| IBIS file stm32h563_573_lqfp144-smps.ibs
[IBIS ver] 4.2
[File name] stm32h563_573_lqfp144-smps.ibs
[File Rev] 1.1
[Date] 07-05-2024
[Source] Data Created at STMicroelectronics
[Notes]  File originated from ELDO simulations.
[Disclaimer]  This information is for modeling purpose only and is
   not guaranteed. The information is subject to change without
   notice.
[Copyright] Copyright 2024 STMicroelectronics Inc.
|   Component stm32h563_573_lqfp144-smps
[Component] stm32h563_573_lqfp144-smps
[Manufacturer] STMicroelectronics
[Package]
| variable   typ   min   max
R_pkg  0  NA  NA
L_pkg  0  NA  NA
C_pkg  0  NA  NA
[Pin]   signal_name   model_name
1  PE2  io8_ft_i3c_spi
2  PE3  io8_ft_i3c_spi
3  PE4  io8_ft_i3c_spi
4  PE5  io8_ft_i3c_spi
5  PE6  io8_ft_i3c_spi
6  VBAT  power
7  PC13  io8_ft_i3c_spi
8  PC14-OSC32_IN  io8_ft_i3c_spi
9  PC15  io8_ft_i3c_spi
10  PF0  io8_ft_i3c_spi
11  PF1  io8_ft_i3c_spi
12  PF2  io8_ft_i3c_spi
13  PF3  io8_ft_i3c_spi
14  PF4  io8_ft_i3c_spi
15  PF5  io8_ft_i3c_spi
16  VSS  gnd
17  VDD  power
18  PF6  io8_ft_i3c_spi
19  PF7  io8_ft_i3c_spi
20  PF8  io8_ft_i3c_spi
21  PF9  io8_ft_i3c_spi
22  PF10  io8_ft_i3c_spi
23  PH0-OSC_IN  io8_ft_i3c_spi
24  PH1-OSC_OUT  io8_ft_i3c_spi
25  NRST  ioreset_ft_v33
26  PC0  io8_ft_spi
27  PC1  io8_ft_spi
28  PC2  io8_ft_spi
29  PC3  io8_ft_spi
30  VSSA  nc
31  VREFP  nc
32  VDDA  nc
33  PA0  io8_ft_spi
34  PA1  io8_ft_spi_tamp
35  PA2  io8_ft_spi
36  PA3  io8_ft_spi
37  VSS  gnd
38  VDD  power
39  PA4  io8_ft_spi
40  PA5  io8_ft_spi
41  PA6  io8_ft_spi
42  PA7  io8_ft_spi
43  PB0  io8_ft_spi
44  PB1  io8_ft_spi
45  PB2  io8_ft_i3c_spi
46  PF11  io8_ft_spi
47  PF12  io8_ft_spi
48  VSS  gnd
49  VDD  power
50  PF13  io8_ft_spi
51  PF14  io8_ft_spi
52  PF15  io8_ft_i3c_spi
53  PG0  io8_ft_i3c_spi
54  PG1  io8_ft_i3c_spi
55  PE7  io8_ft_i3c_spi
56  PE8  io8_ft_i3c_spi
57  PE9  io8_ft_i3c_spi
58  VSS  gnd
59  VDD  power
60  PE10  io8_ft_i3c_spi
61  PE11  io8_ft_i3c_spi
62  PE12  io8_ft_i3c_spi
63  PE13  io8_ft_i3c_spi
64  PE14  io8_ft_i3c_spi
65  PE15  io8_ft_i3c_spi
66  PB10  io8_ft_i3c_spi
67  PB11  io8_ft_i3c_spi
68  VLXSMPS  nc
69  VDDSMPS  nc
70  VSSSMPS  nc
71  VCAP  nc
72  VSS  gnd
73  VDD  power
|74  PB13  io8usb_ft_pd
|75  PB14  io8usb_ft_pd
74  PB13  nc
75  PB14  nc
76  PB15  io8_ft_spi
77  PD8  io8_ft_i3c_spi
78  PD9  io8_ft_i3c_spi
79  PD10  io8_ft_i3c_spi
80  PD11  io8_ft_i3c_spi
81  PD12  io8_ft_i3c_spi
82  PD13  io8_ft_i3c_spi
83  VSS  gnd
84  VDD  power
85  PD14  io8_ft_i3c_spi
86  PD15  io8_ft_i3c_spi
87  PG2  io8_ft_i3c_spi
88  PG3  io8_ft_i3c_spi
89  PG4  io8_ft_i3c_spi
90  PG5  io8_ft_i3c_spi
91  PG6  io8_ft_i3c_spi
92  PG7  io8_ft_i3c_spi
93  PG8  io8_ft_i3c_spi
94  VSS  gnd
95  VDD  power
96  PC6  io8_ft_i3c_spi
97  PC7  io8_ft_i3c_spi
98  PC8  io8_ft_i3c_spi
99  PC9  io8_ft_i3c_spi
100  PA8  io8_ft_i3c_spi
101  PA9  io8_ft_i3c_spi
102  PA10  io8_ft_i3c_spi
103  PA11  io8usb_ft_i3c_spi_phy
104  PA12  io8usb_ft_i3c_spi_phy
105  PA13  io8_ft_i3c_spi
106  VDDUSB  power
107  VSS  gnd
108  VDD  power
109  PA14  io8_ft_i3c_spi
110  PA15  io8_ft_i3c_spi
111  PC10  io8_ft_i3c_spi
112  PC11  io8_ft_i3c_spi
113  PC12  io8_ft_i3c_spi
114  PD0  io8_ft_i3c_spi
115  PD1  io8_ft_i3c_spi
116  PD2  io8_ft_i3c_spi
117  PD3  io8_ft_i3c_spi
118  PD4  io8_ft_i3c_spi
119  PD5  io8_ft_i3c_spi
120  VSS  gnd
121  VDDIO2  power
122  PD6  io8_ft_i3c_spi
123  PD7  io8_ft_i3c_spi
124  PG9  io8_ft_i3c_spi
125  PG10  io8_ft_i3c_spi
126  PG12  io8_ft_i3c_spi
127  PG13  io8_ft_i3c_spi
128  PG14  io8_ft_i3c_spi
129  VSS  gnd
130  VDD  power
131  PG15  io8_ft_i3c_spi
132  PB3  io8_ft_i3c_spi
133  PB4  io8_ft_i3c_spi
134  PB5  io8_ft_i3c_spi
135  PB6  io8_ft_i3c_spi
136  PB7  io8_ft_i3c_spi
137  BOOT0  vpphv
138  PB8  io8_ft_i3c_spi
139  PB9  io8_ft_i3c_spi
140  PE0  io8_ft_i3c_spi
141  PE1  io8_ft_i3c_spi
142  VCAP  nc
143  VSS  gnd
144  VDD  power
[Package Model]   484-lqfp-20x20-144-smps-221014
[Pin Mapping]   pulldown_ref   pullup_ref   | Comment
1  gndio  vddiom
2  gndio  vddiom
3  gndio  vddiom
4  gndio  vddiom
5  gndio  vddiom
6  nc  vsw
7  gndio  vddiom  | Depending on IO usage
| 7  gndio  vsw  | Depending on IO usage
8  gndio  vddiom  | Depending on IO usage
| 8  gndio  vsw  | Depending on IO usage
9  gndio  vddiom  | Depending on IO usage
| 9  gndio  vsw  | Depending on IO usage
10  gndio  vddiom
11  gndio  vddiom
12  gndio  vddiom
13  gndio  vddiom
14  gndio  vddiom
15  gndio  vddiom
16  gndio  nc
17  nc  vddiom
18  gndio  vddiom
19  gndio  vddiom
20  gndio  vddiom
21  gndio  vddiom
22  gndio  vddiom
23  gndio  vddiom
24  gndio  vddiom
25  gndio  vddiom
26  gndio  vddiom
27  gndio  vddiom
28  gndio  vddiom
29  gndio  vddiom
30  nc  nc
31  nc  nc
32  nc  nc
33  gndio  vddiom
34  gndio  vddiom
35  gndio  vddiom
36  gndio  vddiom
37  gndio  nc
38  nc  vddiom
39  gndio  vddiom
40  gndio  vddiom
41  gndio  vddiom
42  gndio  vddiom
43  gndio  vddiom
44  gndio  vddiom
45  gndio  vddiom
46  gndio  vddiom
47  gndio  vddiom
48  gndio  nc
49  nc  vddiom
50  gndio  vddiom
51  gndio  vddiom
52  gndio  vddiom
53  gndio  vddiom
54  gndio  vddiom
55  gndio  vddiom
56  gndio  vddiom
57  gndio  vddiom
58  gndio  nc
59  nc  vddiom
60  gndio  vddiom
61  gndio  vddiom
62  gndio  vddiom
63  gndio  vddiom
64  gndio  vddiom
65  gndio  vddiom
66  gndio  vddiom
67  gndio  vddiom
68  nc  nc
69  nc  nc
70  nc  nc
71  nc  nc
72  gndio  nc
73  nc  vddiom
|74  gndio  vddiom
|75  gndio  vddiom
74 nc nc
75 nc nc
76  gndio  vddiom
77  gndio  vddiom
78  gndio  vddiom
79  gndio  vddiom
80  gndio  vddiom
81  gndio  vddiom
82  gndio  vddiom
83  gndio  nc
84  nc  vddiom
85  gndio  vddiom
86  gndio  vddiom
87  gndio  vddiom
88  gndio  vddiom
89  gndio  vddiom
90  gndio  vddiom
91  gndio  vddiom
92  gndio  vddiom
93  gndio  vddiom
94  gndio  nc
95  nc  vddiom
96  gndio  vddiom
97  gndio  vddiom
98  gndio  vddiom
99  gndio  vddiom
100  gndio  vddiom
101  gndio  vddiom  | Depending on IO usage
| 101  gndio  vddusb  | Depending on IO usage
102  gndio  vddiom  | Depending on IO usage
| 102  gndio  vddusb  | Depending on IO usage
103  gndio  vddiom  | Depending on IO usage
| 103  gndio  vddusb  | Depending on IO usage
104  gndio  vddiom  | Depending on IO usage
| 104  gndio  vddusb  | Depending on IO usage
105  gndio  vddiom  | Depending on IO usage
| 105  gndio  vddusb  | Depending on IO usage
106  nc  vddusb
107  gndio  nc
108  nc  vddiom
109  gndio  vddiom
110  gndio  vddiom
111  gndio  vddiom
112  gndio  vddiom
113  gndio  vddiom
114  gndio  vddiom
115  gndio  vddiom
116  gndio  vddiom
117  gndio  vddiom
118  gndio  vddiom
119  gndio  vddiom
120  gndio  nc
121  nc  vddmmc
122  gndio  vddiom  | Depending on IO usage
| 122  gndio  vddmmc  | Depending on IO usage
123  gndio  vddiom  | Depending on IO usage
| 123  gndio  vddmmc  | Depending on IO usage
124  gndio  vddiom  | Depending on IO usage
| 124  gndio  vddmmc  | Depending on IO usage
125  gndio  vddiom  | Depending on IO usage
| 125  gndio  vddmmc  | Depending on IO usage
126  gndio  vddiom  | Depending on IO usage
| 126  gndio  vddmmc  | Depending on IO usage
127  gndio  vddiom  | Depending on IO usage
| 127  gndio  vddmmc  | Depending on IO usage
128  gndio  vddiom  | Depending on IO usage
| 128  gndio  vddmmc  | Depending on IO usage
129  gndio  nc
130  nc  vddiom
131  gndio  vddiom  | Depending on IO usage
| 131  gndio  vddmmc  | Depending on IO usage
132  gndio  vddiom  | Depending on IO usage
| 132  gndio  vddmmc  | Depending on IO usage
133  gndio  vddiom  | Depending on IO usage
| 133  gndio  vddmmc  | Depending on IO usage
134  gndio  vddiom  | Depending on IO usage
| 134  gndio  vddmmc  | Depending on IO usage
135  gndio  vddiom  | Depending on IO usage
| 135  gndio  vddmmc  | Depending on IO usage
136  gndio  vddiom  | Depending on IO usage
| 136  gndio  vddmmc  | Depending on IO usage
137  gndio  vddiom  | Depending on IO usage
| 137  gndio  vddmmc  | Depending on IO usage
138  gndio  vddiom  | Depending on IO usage
| 138  gndio  vddmmc  | Depending on IO usage
139  gndio  vddiom  | Depending on IO usage
| 139  gndio  vddmmc  | Depending on IO usage
140  gndio  vddiom  | Depending on IO usage
| 140  gndio  vddmmc  | Depending on IO usage
141  gndio  vddiom  | Depending on IO usage
| 141  gndio  vddmmc  | Depending on IO usage
142  nc  nc
143  gndio  nc
144  nc  vddiom
[Model Selector] io8_ft_i3c_spi
io8_ft_spi_ls_1v2 "io8_ft spi low speed @ 1.2V"
io8_ft_spi_ls_1v8 "io8_ft spi low speed @ 1.8V"
io8_ft_spi_ls_3v3 "io8_ft spi low speed @ 3.3V"
io8_ft_spi_ms_1v2 "io8_ft spi med speed @ 1.2V"
io8_ft_spi_ms_1v8 "io8_ft spi med speed @ 1.8V"
io8_ft_spi_ms_3v3 "io8_ft spi med speed @ 3.3V"
io8_ft_spi_fs_1v2 "io8_ft spi fast speed @ 1.2V"
io8_ft_spi_fs_1v8 "io8_ft spi fast speed @ 1.8V"
io8_ft_spi_fs_3v3 "io8_ft spi fast speed @ 3.3V"
io8_ft_spi_hs_1v2 "io8_ft spi high speed @ 1.2V"
io8_ft_spi_hs_1v8 "io8_ft spi high speed @ 1.8V"
io8_ft_spi_hs_3v3 "io8_ft spi high speed @ 3.3V"
io8_ft_hslv_spi_ls_1v2 "io8_ft spi hslv low speed @ 1.2V"
io8_ft_hslv_spi_ls_1v8 "io8_ft spi hslv low speed @ 1.8V"
io8_ft_hslv_spi_ls_2v5 "io8_ft spi hslv low speed @ 2.5V"
io8_ft_hslv_spi_ms_1v2 "io8_ft spi hslv med speed @ 1.2V"
io8_ft_hslv_spi_ms_1v8 "io8_ft spi hslv med speed @ 1.8V"
io8_ft_hslv_spi_ms_2v5 "io8_ft spi hslv med speed @ 2.5V"
io8_ft_hslv_spi_fs_1v2 "io8_ft spi hslv fast speed @ 1.2V"
io8_ft_hslv_spi_fs_1v8 "io8_ft spi hslv fast speed @ 1.8V"
io8_ft_hslv_spi_fs_2v5 "io8_ft spi hslv fast speed @ 2.5V"
io8_ft_hslv_spi_hs_1v2 "io8_ft spi hslv high speed @ 1.2V"
io8_ft_hslv_spi_hs_1v8 "io8_ft spi hslv high speed @ 1.8V"
io8_ft_hslv_spi_hs_2v5 "io8_ft spi hslv high speed @ 2.5V"
io8_ft_i3c_spi_ls_1v2 "io8_ft i3c spi open-drain low speed @ 1.2V"
io8_ft_i3c_spi_ls_1v8 "io8_ft i3c spi open-drain low speed @ 1.8V"
io8_ft_i3c_spi_ls_3v3 "io8_ft i3c spi open-drain low speed @ 3.3V"
io8_ft_i3c_spi_ms_1v2 "io8_ft i3c spi open-drain med speed @ 1.2V"
io8_ft_i3c_spi_ms_1v8 "io8_ft i3c spi open-drain med speed @ 1.8V"
io8_ft_i3c_spi_ms_3v3 "io8_ft i3c spi open-drain med speed @ 3.3V"
io8_ft_i3c_spi_fs_1v2 "io8_ft i3c spi open-drain fast speed @ 1.2V"
io8_ft_i3c_spi_fs_1v8 "io8_ft i3c spi open-drain fast speed @ 1.8V"
io8_ft_i3c_spi_fs_3v3 "io8_ft i3c spi open-drain fast speed @ 3.3V"
io8_ft_i3c_spi_hs_1v2 "io8_ft i3c spi open-drain high speed @ 1.2V"
io8_ft_i3c_spi_hs_1v8 "io8_ft i3c spi open-drain high speed @ 1.8V"
io8_ft_i3c_spi_hs_3v3 "io8_ft i3c spi open-drain high speed @ 3.3V"
io8_ft_hslv_i3c_spi_ls_1v2 "io8_ft hslv i3c spi open-drain low speed @ 1.2V"
io8_ft_hslv_i3c_spi_ls_1v8 "io8_ft hslv i3c spi open-drain low speed @ 1.8V"
io8_ft_hslv_i3c_spi_ls_2v5 "io8_ft hslv i3c spi open-drain low speed @ 2.5V"
io8_ft_hslv_i3c_spi_ms_1v2 "io8_ft hslv i3c spi open-drain med speed @ 1.2V"
io8_ft_hslv_i3c_spi_ms_1v8 "io8_ft hslv i3c spi open-drain med speed @ 1.8V"
io8_ft_hslv_i3c_spi_ms_2v5 "io8_ft hslv i3c spi open-drain med speed @ 2.5V"
io8_ft_hslv_i3c_spi_fs_1v2 "io8_ft hslv i3c spi open-drain fast speed @ 1.2V"
io8_ft_hslv_i3c_spi_fs_1v8 "io8_ft hslv i3c spi open-drain fast speed @ 1.8V"
io8_ft_hslv_i3c_spi_fs_2v5 "io8_ft hslv i3c spi open-drain fast speed @ 2.5V"
io8_ft_hslv_i3c_spi_hs_1v2 "io8_ft hslv i3c spi open-drain high speed @ 1.2V"
io8_ft_hslv_i3c_spi_hs_1v8 "io8_ft hslv i3c spi open-drain high speed @ 1.8V"
io8_ft_hslv_i3c_spi_hs_2v5 "io8_ft hslv i3c spi open-drain high speed @ 2.5V"
io8_ft_i3c_fmp_spi_3v3 "io8_ft i3c fm+ spi open-drain @ 3.3V"
io8_ft_i3c_fmp_spi_1v8 "io8_ft i3c fm+ spi open-drain @ 1.8V"
io8_ft_i3c_fmp_spi_1v2 "io8_ft i3c fm+ spi open-drain @ 1.2V"
[Model Selector] io8_ft_spi
io8_ft_spi_ls_1v2 "io8_ft spi low speed @ 1.2V"
io8_ft_spi_ls_1v8 "io8_ft spi low speed @ 1.8V"
io8_ft_spi_ls_3v3 "io8_ft spi low speed @ 3.3V"
io8_ft_spi_ms_1v2 "io8_ft spi med speed @ 1.2V"
io8_ft_spi_ms_1v8 "io8_ft spi med speed @ 1.8V"
io8_ft_spi_ms_3v3 "io8_ft spi med speed @ 3.3V"
io8_ft_spi_fs_1v2 "io8_ft spi fast speed @ 1.2V"
io8_ft_spi_fs_1v8 "io8_ft spi fast speed @ 1.8V"
io8_ft_spi_fs_3v3 "io8_ft spi fast speed @ 3.3V"
io8_ft_spi_hs_1v2 "io8_ft spi high speed @ 1.2V"
io8_ft_spi_hs_1v8 "io8_ft spi high speed @ 1.8V"
io8_ft_spi_hs_3v3 "io8_ft spi high speed @ 3.3V"
io8_ft_hslv_spi_ls_1v2 "io8_ft spi hslv low speed @ 1.2V"
io8_ft_hslv_spi_ls_1v8 "io8_ft spi hslv low speed @ 1.8V"
io8_ft_hslv_spi_ls_2v5 "io8_ft spi hslv low speed @ 2.5V"
io8_ft_hslv_spi_ms_1v2 "io8_ft spi hslv med speed @ 1.2V"
io8_ft_hslv_spi_ms_1v8 "io8_ft spi hslv med speed @ 1.8V"
io8_ft_hslv_spi_ms_2v5 "io8_ft spi hslv med speed @ 2.5V"
io8_ft_hslv_spi_fs_1v2 "io8_ft spi hslv fast speed @ 1.2V"
io8_ft_hslv_spi_fs_1v8 "io8_ft spi hslv fast speed @ 1.8V"
io8_ft_hslv_spi_fs_2v5 "io8_ft spi hslv fast speed @ 2.5V"
io8_ft_hslv_spi_hs_1v2 "io8_ft spi hslv high speed @ 1.2V"
io8_ft_hslv_spi_hs_1v8 "io8_ft spi hslv high speed @ 1.8V"
io8_ft_hslv_spi_hs_2v5 "io8_ft spi hslv high speed @ 2.5V"
[Model Selector] io8_ft_spi_tamp
io8_ft_spi_ls_1v2 "io8_ft spi low speed @ 1.2V"
io8_ft_spi_ls_1v8 "io8_ft spi low speed @ 1.8V"
io8_ft_spi_ls_3v3 "io8_ft spi low speed @ 3.3V"
io8_ft_spi_ms_1v2 "io8_ft spi med speed @ 1.2V"
io8_ft_spi_ms_1v8 "io8_ft spi med speed @ 1.8V"
io8_ft_spi_ms_3v3 "io8_ft spi med speed @ 3.3V"
io8_ft_spi_fs_1v2 "io8_ft spi fast speed @ 1.2V"
io8_ft_spi_fs_1v8 "io8_ft spi fast speed @ 1.8V"
io8_ft_spi_fs_3v3 "io8_ft spi fast speed @ 3.3V"
io8_ft_spi_hs_1v2 "io8_ft spi high speed @ 1.2V"
io8_ft_spi_hs_1v8 "io8_ft spi high speed @ 1.8V"
io8_ft_spi_hs_3v3 "io8_ft spi high speed @ 3.3V"
io8_ft_hslv_spi_ls_1v2 "io8_ft spi hslv low speed @ 1.2V"
io8_ft_hslv_spi_ls_1v8 "io8_ft spi hslv low speed @ 1.8V"
io8_ft_hslv_spi_ls_2v5 "io8_ft spi hslv low speed @ 2.5V"
io8_ft_hslv_spi_ms_1v2 "io8_ft spi hslv med speed @ 1.2V"
io8_ft_hslv_spi_ms_1v8 "io8_ft spi hslv med speed @ 1.8V"
io8_ft_hslv_spi_ms_2v5 "io8_ft spi hslv med speed @ 2.5V"
io8_ft_hslv_spi_fs_1v2 "io8_ft spi hslv fast speed @ 1.2V"
io8_ft_hslv_spi_fs_1v8 "io8_ft spi hslv fast speed @ 1.8V"
io8_ft_hslv_spi_fs_2v5 "io8_ft spi hslv fast speed @ 2.5V"
io8_ft_hslv_spi_hs_1v2 "io8_ft spi hslv high speed @ 1.2V"
io8_ft_hslv_spi_hs_1v8 "io8_ft spi hslv high speed @ 1.8V"
io8_ft_hslv_spi_hs_2v5 "io8_ft spi hslv high speed @ 2.5V"
io8_ft_tamp_v33_1v2 "io8_ft tamp V33 @ 1.2V"
io8_ft_tamp_v33_1v8 "io8_ft tamp V33 @ 1.2V"
io8_ft_tamp_v33_3v3 "io8_ft tamp V33 @ 1.2V"
[Model Selector] io8usb_ft_i3c_spi_phy
io8_ft_spi_ls_1v2 "io8_ft spi low speed @ 1.2V"
io8_ft_spi_ls_1v8 "io8_ft spi low speed @ 1.8V"
io8_ft_spi_ls_3v3 "io8_ft spi low speed @ 3.3V"
io8_ft_spi_ms_1v2 "io8_ft spi med speed @ 1.2V"
io8_ft_spi_ms_1v8 "io8_ft spi med speed @ 1.8V"
io8_ft_spi_ms_3v3 "io8_ft spi med speed @ 3.3V"
io8_ft_spi_fs_1v2 "io8_ft spi fast speed @ 1.2V"
io8_ft_spi_fs_1v8 "io8_ft spi fast speed @ 1.8V"
io8_ft_spi_fs_3v3 "io8_ft spi fast speed @ 3.3V"
io8_ft_spi_hs_1v2 "io8_ft spi high speed @ 1.2V"
io8_ft_spi_hs_1v8 "io8_ft spi high speed @ 1.8V"
io8_ft_spi_hs_3v3 "io8_ft spi high speed @ 3.3V"
io8_ft_hslv_spi_ls_1v2 "io8_ft spi hslv low speed @ 1.2V"
io8_ft_hslv_spi_ls_1v8 "io8_ft spi hslv low speed @ 1.8V"
io8_ft_hslv_spi_ls_2v5 "io8_ft spi hslv low speed @ 2.5V"
io8_ft_hslv_spi_ms_1v2 "io8_ft spi hslv med speed @ 1.2V"
io8_ft_hslv_spi_ms_1v8 "io8_ft spi hslv med speed @ 1.8V"
io8_ft_hslv_spi_ms_2v5 "io8_ft spi hslv med speed @ 2.5V"
io8_ft_hslv_spi_fs_1v2 "io8_ft spi hslv fast speed @ 1.2V"
io8_ft_hslv_spi_fs_1v8 "io8_ft spi hslv fast speed @ 1.8V"
io8_ft_hslv_spi_fs_2v5 "io8_ft spi hslv fast speed @ 2.5V"
io8_ft_hslv_spi_hs_1v2 "io8_ft spi hslv high speed @ 1.2V"
io8_ft_hslv_spi_hs_1v8 "io8_ft spi hslv high speed @ 1.8V"
io8_ft_hslv_spi_hs_2v5 "io8_ft spi hslv high speed @ 2.5V"
io8_ft_i3c_spi_ls_1v2 "io8_ft i3c spi open-drain low speed @ 1.2V"
io8_ft_i3c_spi_ls_1v8 "io8_ft i3c spi open-drain low speed @ 1.8V"
io8_ft_i3c_spi_ls_3v3 "io8_ft i3c spi open-drain low speed @ 3.3V"
io8_ft_i3c_spi_ms_1v2 "io8_ft i3c spi open-drain med speed @ 1.2V"
io8_ft_i3c_spi_ms_1v8 "io8_ft i3c spi open-drain med speed @ 1.8V"
io8_ft_i3c_spi_ms_3v3 "io8_ft i3c spi open-drain med speed @ 3.3V"
io8_ft_i3c_spi_fs_1v2 "io8_ft i3c spi open-drain fast speed @ 1.2V"
io8_ft_i3c_spi_fs_1v8 "io8_ft i3c spi open-drain fast speed @ 1.8V"
io8_ft_i3c_spi_fs_3v3 "io8_ft i3c spi open-drain fast speed @ 3.3V"
io8_ft_i3c_spi_hs_1v2 "io8_ft i3c spi open-drain high speed @ 1.2V"
io8_ft_i3c_spi_hs_1v8 "io8_ft i3c spi open-drain high speed @ 1.8V"
io8_ft_i3c_spi_hs_3v3 "io8_ft i3c spi open-drain high speed @ 3.3V"
io8_ft_hslv_i3c_spi_ls_1v2 "io8_ft hslv i3c spi open-drain low speed @ 1.2V"
io8_ft_hslv_i3c_spi_ls_1v8 "io8_ft hslv i3c spi open-drain low speed @ 1.8V"
io8_ft_hslv_i3c_spi_ls_2v5 "io8_ft hslv i3c spi open-drain low speed @ 2.5V"
io8_ft_hslv_i3c_spi_ms_1v2 "io8_ft hslv i3c spi open-drain med speed @ 1.2V"
io8_ft_hslv_i3c_spi_ms_1v8 "io8_ft hslv i3c spi open-drain med speed @ 1.8V"
io8_ft_hslv_i3c_spi_ms_2v5 "io8_ft hslv i3c spi open-drain med speed @ 2.5V"
io8_ft_hslv_i3c_spi_fs_1v2 "io8_ft hslv i3c spi open-drain fast speed @ 1.2V"
io8_ft_hslv_i3c_spi_fs_1v8 "io8_ft hslv i3c spi open-drain fast speed @ 1.8V"
io8_ft_hslv_i3c_spi_fs_2v5 "io8_ft hslv i3c spi open-drain fast speed @ 2.5V"
io8_ft_hslv_i3c_spi_hs_1v2 "io8_ft hslv i3c spi open-drain high speed @ 1.2V"
io8_ft_hslv_i3c_spi_hs_1v8 "io8_ft hslv i3c spi open-drain high speed @ 1.8V"
io8_ft_hslv_i3c_spi_hs_2v5 "io8_ft hslv i3c spi open-drain high speed @ 2.5V"
io8_ft_i3c_fmp_spi_3v3 "io8_ft i3c fm+ spi open-drain @ 3.3V"
io8_ft_i3c_fmp_spi_1v8 "io8_ft i3c fm+ spi open-drain @ 1.8V"
io8_ft_i3c_fmp_spi_1v2 "io8_ft i3c fm+ spi open-drain @ 1.2V"
io8usb_ft_phy_ls_2v5 "iousb ft low speed @ 2.5V"
io8usb_ft_phy_ls_3v3 "iousb ft low speed @ 3.3V"
io8usb_ft_phy_fs_2v5 "iousb ft fast speed @ 2.5V"
io8usb_ft_phy_fs_3v3 "iousb ft fast speed @ 3.3V"
[Model Selector] ioreset_ft_v33
ioreset_ft_v33_1v2 "Reset PAD. 5V tolerant. 1.2V range"
ioreset_ft_v33_1v8 "Reset PAD. 5V tolerant. 1.8V range"
ioreset_ft_v33_3v3 "Reset PAD. 5V tolerant. 3.3V range"
[Model Selector] vpphv
vpphv_1v2 "Flash Test cell v33 = 1.2 V range"
vpphv_1v8 "Flash Test cell v33 = 1.8 V range"
vpphv_3v3 "Flash Test cell v33 = 3.3 V range"
[Define Package Model]  484-lqfp-20x20-144-smps-221014
[Manufacturer]  Unknown
[OEM]  Unknown
[Description]  None
[Number Of Pins]  137
[Pin Numbers]
| Pin Num   Terminal Name
137 | BOOT0
25 | NRST
33 | PA0
34 | PA1
35 | PA2
36 | PA3
39 | PA4
40 | PA5
41 | PA6
42 | PA7
100 | PA8
101 | PA9
102 | PA10
103 | PA11
104 | PA12
105 | PA13
109 | PA14
110 | PA15
43 | PB0
44 | PB1
45 | PB2
132 | PB3
133 | PB4
134 | PB5
135 | PB6
136 | PB7
138 | PB8
139 | PB9
66 | PB10
67 | PB11
74 | PB13
75 | PB14
76 | PB15
26 | PC0
27 | PC1
28 | PC2
29 | PC3
96 | PC6
97 | PC7
98 | PC8
99 | PC9
111 | PC10
112 | PC11
113 | PC12
7 | PC13
8 | PC14-OSC32_IN
9 | PC15-OSC32_OUT
114 | PD0
115 | PD1
116 | PD2
117 | PD3
118 | PD4
119 | PD5
122 | PD6
123 | PD7
77 | PD8
78 | PD9
79 | PD10
80 | PD11
81 | PD12
82 | PD13
85 | PD14
86 | PD15
140 | PE0
141 | PE1
1 | PE2
2 | PE3
3 | PE4
4 | PE5
5 | PE6
55 | PE7
56 | PE8
57 | PE9
60 | PE10
61 | PE11
62 | PE12
63 | PE13
64 | PE14
65 | PE15
10 | PF0
11 | PF1
12 | PF2
13 | PF3
14 | PF4
15 | PF5
18 | PF6
19 | PF7
20 | PF8
21 | PF9
22 | PF10
46 | PF11
47 | PF12
50 | PF13
51 | PF14
52 | PF15
53 | PG0
54 | PG1
87 | PG2
88 | PG3
89 | PG4
90 | PG5
91 | PG6
92 | PG7
93 | PG8
124 | PG9
125 | PG10
126 | PG12
127 | PG13
128 | PG14
131 | PG15
23 | PH0-OSC_IN
24 | PH1-OSC_OUT
6 | VBAT
71 | VCAP
142 | VCAP
73 | VDD
108 | VDD
17 | VDD
38 | VDD
49 | VDD
59 | VDD
144 | VDD
84 | VDD
130 | VDD
95 | VDD
121 | VDDIO2
106 | VDDUSB
32 | VDDA
69 | VDDSMPS
68 | VLXSMPS
31 | VREFP
48 | VSS
129 | VSS
94 | VSS
16 | VSS
30 | VSSA
70 | VSSSMPS
|[Merged Pins]  16
|37  |  VSS
|58  |  VSS
|72  |  VSS
|83  |  VSS
|107  |  VSS
|120  |  VSS
|143  |  VSS
[Model Data]
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[End Model Data]
[End Package Model]
|End [Component]
| Models and submodels in the file (64): io8_ft_hslv_i3c_spi_fs_1v2 (I/O_open_drain), io8_ft_hslv_i3c_spi_fs_1v8 (I/O_open_drain), io8_ft_hslv_i3c_spi_fs_2v5 (I/O_open_drain), io8_ft_hslv_i3c_spi_hs_1v2 (I/O_open_drain), io8_ft_hslv_i3c_spi_hs_1v8 (I/O_open_drain), io8_ft_hslv_i3c_spi_hs_2v5 (I/O_open_drain), io8_ft_hslv_i3c_spi_ls_1v2 (I/O_open_drain), io8_ft_hslv_i3c_spi_ls_1v8 (I/O_open_drain), io8_ft_hslv_i3c_spi_ls_2v5 (I/O_open_drain), io8_ft_hslv_i3c_spi_ms_1v2 (I/O_open_drain), io8_ft_hslv_i3c_spi_ms_1v8 (I/O_open_drain), io8_ft_hslv_i3c_spi_ms_2v5 (I/O_open_drain), io8_ft_hslv_spi_fs_1v2 (I/O), io8_ft_hslv_spi_fs_1v8 (I/O), io8_ft_hslv_spi_fs_2v5 (I/O), io8_ft_hslv_spi_hs_1v2 (I/O), io8_ft_hslv_spi_hs_1v8 (I/O), io8_ft_hslv_spi_hs_2v5 (I/O), io8_ft_hslv_spi_ls_1v2 (I/O), io8_ft_hslv_spi_ls_1v8 (I/O), io8_ft_hslv_spi_ls_2v5 (I/O), io8_ft_hslv_spi_ms_1v2 (I/O), io8_ft_hslv_spi_ms_1v8 (I/O), io8_ft_hslv_spi_ms_2v5 (I/O), io8_ft_i3c_fmp_spi_1v2 (I/O_open_drain), io8_ft_i3c_fmp_spi_1v8 (I/O_open_drain), io8_ft_i3c_fmp_spi_3v3 (I/O_open_drain), io8_ft_i3c_spi_fs_1v2 (I/O_open_drain), io8_ft_i3c_spi_fs_1v8 (I/O_open_drain), io8_ft_i3c_spi_fs_3v3 (I/O_open_drain), io8_ft_i3c_spi_hs_1v2 (I/O_open_drain), io8_ft_i3c_spi_hs_1v8 (I/O_open_drain), io8_ft_i3c_spi_hs_3v3 (I/O_open_drain), io8_ft_i3c_spi_ls_1v2 (I/O_open_drain), io8_ft_i3c_spi_ls_1v8 (I/O_open_drain), io8_ft_i3c_spi_ls_3v3 (I/O_open_drain), io8_ft_i3c_spi_ms_1v2 (I/O_open_drain), io8_ft_i3c_spi_ms_1v8 (I/O_open_drain), io8_ft_i3c_spi_ms_3v3 (I/O_open_drain), io8_ft_spi_fs_1v2 (I/O), io8_ft_spi_fs_1v8 (I/O), io8_ft_spi_fs_3v3 (I/O), io8_ft_spi_hs_1v2 (I/O), io8_ft_spi_hs_1v8 (I/O), io8_ft_spi_hs_3v3 (I/O), io8_ft_spi_ls_1v2 (I/O), io8_ft_spi_ls_1v8 (I/O), io8_ft_spi_ls_3v3 (I/O), io8_ft_spi_ms_1v2 (I/O), io8_ft_spi_ms_1v8 (I/O), io8_ft_spi_ms_3v3 (I/O), io8_ft_tamp_v33_1v2 (I/O), io8_ft_tamp_v33_1v8 (I/O), io8_ft_tamp_v33_3v3 (I/O), io8usb_ft_phy_fs_2v5 (I/O), io8usb_ft_phy_fs_3v3 (I/O), io8usb_ft_phy_ls_2v5 (I/O), io8usb_ft_phy_ls_3v3 (I/O), ioreset_ft_v33_1v2 (I/O_open_drain), ioreset_ft_v33_1v8 (I/O_open_drain), ioreset_ft_v33_3v3 (I/O_open_drain), vpphv_1v2 (Input), vpphv_1v8 (Input), vpphv_3v3 (Input)
